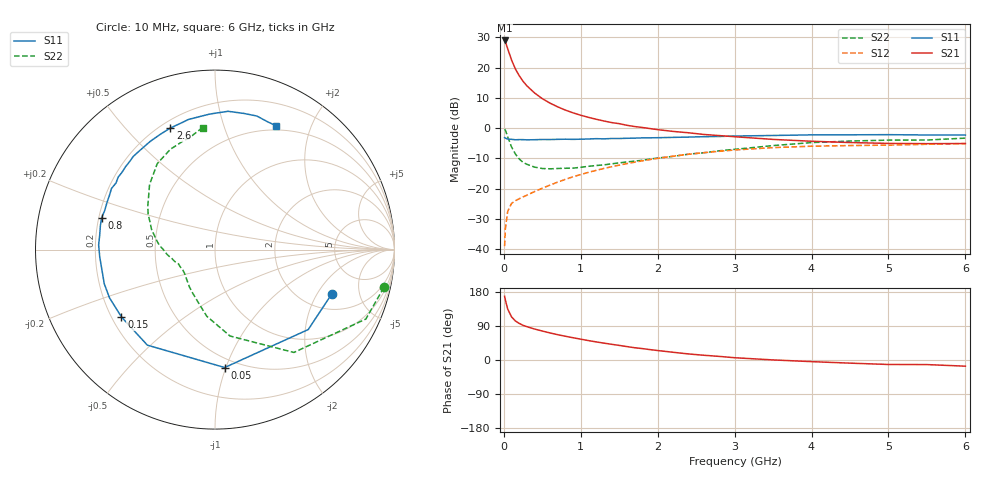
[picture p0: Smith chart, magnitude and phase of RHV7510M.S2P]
! SIEMENS Small Signal Semiconductors
! BFR106
! Si NPN RF Bipolar Junction Transistor in SOT23
! VCE = 0.75 V  IC = 10 mA
! Common Emitter S-Parameters:  August  1996
# GHz  S  MA  R  50
!  f  S11  S21  S12  S22
! GHz  MAG  ANG  MAG  ANG  MAG  ANG  MAG  ANG
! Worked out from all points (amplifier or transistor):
!   36 points, 10 MHz to 6 GHz, reference 50 ohm
!   highest |S21| = 29.0 dB at 10 MHz (marker M1)
!   |S21| within 3 dB of that: start of sweep to 53.69 MHz
!   unconditionally stable (mu >= 1): 447.8 MHz to end of sweep
!   at 250 MHz: K = 0.73, MSG = 19.1 dB, |S12| = -22.7 dB
!   at 1.4 GHz: K = 1.13, MAG = 5.1 dB, |S12| = -12.8 dB
!   at 6 GHz: K = 1.03, MAG = -1.1 dB, |S12| = -5.1 dB
!   S11 on the Smith chart (normalised r, x): 10 MHz: 2.80, -2.69; 50 MHz: 0.43, -0.99; 150 MHz: 0.24, -0.31; 800 MHz: 0.21, +0.13; 2.6 GHz: 0.24, +0.67; 6 GHz: 0.45, +1.52
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0.01  0.6956 -20.9  28.11 168.1  0.0112 81.4  0.9642 -12.6
0.02  0.6843 -40.6  26.8 158.2  0.0218 72.5  0.9253 -24.7
0.05  0.6593 -85.3  20.54 134.4  0.0421 53.9  0.7223 -52.5
0.1  0.6522 -125.3  13.4 113.9  0.0569 41.5  0.4889 -80.1
0.15  0.6423 -144.2  9.504 103.0  0.063 38.7  0.3743 -97.0
0.2  0.6463 -155.4  7.357 96.6  0.0681 38.9  0.309 -107.6
0.25  0.6457 -162.8  5.939 91.5  0.073 40.4  0.2713 -117.5
0.3  0.6404 -168.3  4.995 87.9  0.078 42.9  0.2524 -124.3
0.4  0.6435 -176.4  3.805 81.7  0.0895 46.6  0.2268 -134.7
0.5  0.6488 177.7  3.07 76.4  0.1015 49.3  0.2151 -142.1
0.6  0.6476 172.6  2.589 71.4  0.1144 51.3  0.2125 -147.1
0.7  0.6526 168.0  2.248 66.8  0.1282 52.8  0.2152 -151.4
0.8  0.656 164.3  1.986 62.7  0.1424 53.5  0.2171 -155.5
1.1  0.661 152.9  1.507 51.2  0.1858 53.7  0.2339 -163.6
1.3  0.6647 146.1  1.313 44.5  0.2156 52.3  0.2472 -169.2
1.6  0.6794 137.2  1.114 35.4  0.2593 49.6  0.2762 -176.5
2.2  0.7031 120.7  0.883 20.4  0.3437 41.4  0.3416 168.1
2.6  0.7219 110.1  0.786 12.5  0.3928 35.0  0.392 157.3
3.5  0.7558 92.2  0.651 0.2  0.4764 20.3  0.5145 135.1
4.5  0.7755 78.1  0.578 -8.3  0.5152 5.6  0.6117 114.0
5.5  0.7701 67.7  0.554 -12.1  0.5406 -3.3  0.6357 103.6
6  0.769 63.6  0.556 -16.3  0.5563 -9.7  0.6837 95.8
